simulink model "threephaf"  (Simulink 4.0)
settings: Solver=ode23  StartTime=-eps  StopTime=0.1  FixedStep=0.000001  MaxStep=2e-5  RelTol=1e-3
undefined symbols (not defined in the file or in its folder): Cdc, di, Element, L, R, sfunxy, Symmetrized, Tf, Ts, Udc, Upp, Warning, Yes
libraries: simulink3 x7
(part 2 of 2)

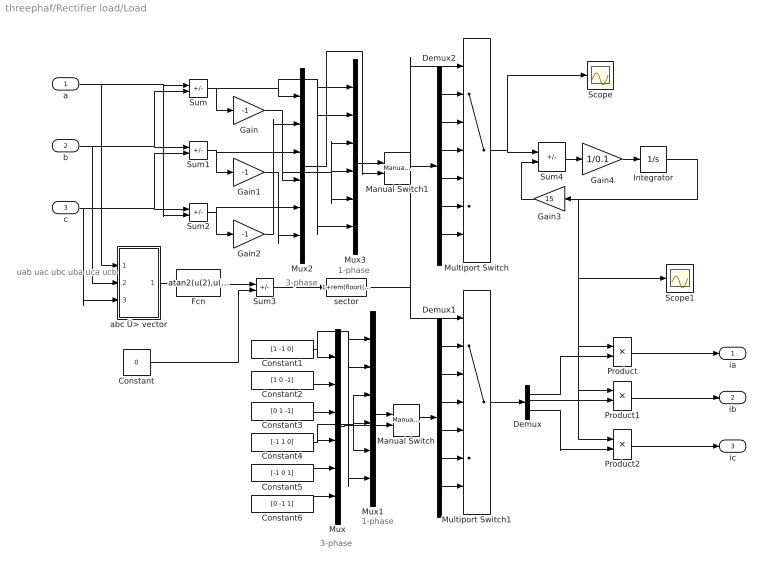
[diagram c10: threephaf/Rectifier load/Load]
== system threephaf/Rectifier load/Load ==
  note: uab uac ubc uba uca ucb
  note: 1-phase
  note: 3-phase
  note: 3-phase
  note: 1-phase
  a : Inport  Port=1  PortDimensions=-1  SampleTime=-1  DataType=auto
  b : Inport  Port=2  PortDimensions=-1  SampleTime=-1  DataType=auto
  c : Inport  Port=3  PortDimensions=-1  SampleTime=-1  DataType=auto
  Constant : Constant  Value=0
  Constant1 : Constant  Value=[1 -1 0]
  Constant2 : Constant  Value=[1 0 -1]
  Constant3 : Constant  Value=[0 1 -1]
  Constant4 : Constant  Value=[-1 1 0]
  Constant5 : Constant  Value=[-1 0 1]
  Constant6 : Constant  Value=[0 -1 1]
  Demux : Demux  Outputs=3  BusSelectionMode=off
  Demux1 : Demux  Outputs=6  BusSelectionMode=off
  Demux2 : Demux  Outputs=6  BusSelectionMode=off
  Fcn : Fcn  Expr=atan2(u(2),u(1))
  Gain : Gain  Gain=-1  Multiplication=Element-wise(K.*u)  SaturateOnIntegerOverflow=on
  Gain1 : Gain  Gain=-1  Multiplication=Element-wise(K.*u)  SaturateOnIntegerOverflow=on
  Gain2 : Gain  Gain=-1  Multiplication=Element-wise(K.*u)  SaturateOnIntegerOverflow=on
  Gain3 : Gain  Orientation=left  Gain=15  Multiplication=Element-wise(K.*u)  SaturateOnIntegerOverflow=on
  Gain4 : Gain  Gain=1/0.1  Multiplication=Element-wise(K.*u)  SaturateOnIntegerOverflow=on
  Integrator : Integrator  ExternalReset=none  InitialConditionSource=internal  InitialCondition=400*sqrt(2)*3/pi/50  LimitOutput=off  UpperSaturationLimit=inf  LowerSaturationLimit=-inf  ShowSaturationPort=off  ShowStatePort=off  AbsoluteTolerance=auto
  Manual Switch : simulink3/Nonlinear/Manual Switch  sw=0  action=0
  Manual Switch1 : simulink3/Nonlinear/Manual Switch  sw=0  action=0
  Multiport Switch : MultiPortSwitch  Inputs=6
  Multiport Switch1 : MultiPortSwitch  Inputs=6
  Mux{,1..3} (4 alike) : Mux  Inputs=6
  Product : Product  Inputs=2  Multiplication=Element-wise(.*)  SaturateOnIntegerOverflow=on
  Product1 : Product  Inputs=2  Multiplication=Element-wise(.*)  SaturateOnIntegerOverflow=on
  Product2 : Product  Inputs=2  Multiplication=Element-wise(.*)  SaturateOnIntegerOverflow=on
  Scope : Scope
  Scope1 : Scope
  Sum{,1..4} (5 alike) : Sum  Inputs=+-  SaturateOnIntegerOverflow=on
  abc Ü> vector : Subsystem  SimViewingDevice=off
  sector : Fcn  Expr=1+rem(floor((2*pi+u(1)+pi/3)/(pi/3+eps)),6)
  ia : Outport  Port=1  InitialOutput=0
  ib : Outport  Port=2  InitialOutput=0
  ic : Outport  Port=3  InitialOutput=0
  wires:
  Demux/3 -> Product2/2
  Demux/1 -> Product/2
  a/1 -> Sum/1, Sum2/2, abc Ü> vector/1(a)
  b/1 -> Sum1/1, Sum/2, abc Ü> vector/2(b)
  c/1 -> Sum2/1, Sum1/2, abc Ü> vector/3(c)
  Sum/1 -> Mux2/1, Mux3/2, Mux3/6, Mux3/1, Gain/1
  Sum1/1 -> Gain1/1, Mux2/3
  Sum2/1 -> Gain2/1, Mux2/5
  abc Ü> vector/1(vect) -> Fcn/1
  sector/1 -> Multiport Switch/1, Multiport Switch1/1
  Fcn/1 -> Sum3/1
  Sum3/1 -> sector/1
  Constant/1 -> Sum3/2
  Multiport Switch/1 -> Sum4/1, Scope/1
  Gain4/1 -> Integrator/1
  Gain3/1 -> Sum4/2
  Multiport Switch1/1 -> Demux/1
  Demux/2 -> Product1/2
  Product/1 -> ia/1
  Product1/1 -> ib/1
  Product2/1 -> ic/1
  Sum4/1 -> Gain4/1
  Integrator/1 -> Gain3/1, Product/1, Product1/1, Product2/1, Scope1/1
  Demux1/1 -> Multiport Switch1/2
  Demux1/2 -> Multiport Switch1/3
  Demux1/3 -> Multiport Switch1/4
  Demux1/4 -> Multiport Switch1/5
  Demux1/5 -> Multiport Switch1/6
  Demux1/6 -> Multiport Switch1/7
  Constant1/1 -> Mux/1, Mux1/2, Mux1/6, Mux1/1
  Constant2/1 -> Mux/2
  Constant3/1 -> Mux/3
  Constant4/1 -> Mux1/3, Mux1/4, Mux1/5, Mux/4
  Constant5/1 -> Mux/5
  Constant6/1 -> Mux/6
  Mux/1 -> Manual Switch/2
  Manual Switch/1 -> Demux1/1
  Mux1/1 -> Manual Switch/1
  Gain/1 -> Mux2/4, Mux3/3, Mux3/5, Mux3/4
  Gain1/1 -> Mux2/6
  Gain2/1 -> Mux2/2
  Demux2/1 -> Multiport Switch/2
  Demux2/2 -> Multiport Switch/3
  Demux2/3 -> Multiport Switch/4
  Demux2/4 -> Multiport Switch/5
  Demux2/5 -> Multiport Switch/6
  Demux2/6 -> Multiport Switch/7
  Mux3/1 -> Manual Switch1/1
  Manual Switch1/1 -> Demux2/1
  Mux2/1 -> Manual Switch1/2

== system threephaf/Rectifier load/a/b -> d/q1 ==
  vect : Inport  Port=1  PortDimensions=-1  SampleTime=-1  DataType=auto
  angle : Inport  Port=2  PortDimensions=-1  SampleTime=-1  DataType=auto
  Fcn_x : Fcn  Expr=u[1]*cos(u[3])-u[2]*sin(u[3])
  Fcn_y : Fcn  Expr=u[1]*sin(u[3])+u[2]*cos(u[3])
  Mux : Mux  Inputs=2
  Mux1 : Mux  Inputs=2
  Out : Outport  Port=1  InitialOutput=0
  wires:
  Mux1/1 -> Out/1
  Fcn_y/1 -> Mux1/2
  Fcn_x/1 -> Mux1/1
  Mux/1 -> Fcn_y/1, Fcn_x/1
  angle/1 -> Mux/2
  vect/1 -> Mux/1

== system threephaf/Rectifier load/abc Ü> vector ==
  a : Inport  Port=1  PortDimensions=-1  SampleTime=-1  DataType=auto
  b : Inport  Port=2  PortDimensions=-1  SampleTime=-1  DataType=auto
  c : Inport  Port=3  PortDimensions=-1  SampleTime=-1  DataType=auto
  Fcn : Fcn  Expr=sqrt(3/2)*u[1]
  Fcn1 : Fcn  Expr=sqrt(1/2)*(u[1]-u[2])
  Gain : Gain  Gain=1/3  Multiplication=Element-wise(K.*u)  SaturateOnIntegerOverflow=on
  Mux5 : Mux  Inputs=2
  Mux7 : Mux  Inputs=2
  Sum2 : Sum  Inputs=+++  SaturateOnIntegerOverflow=on
  Ü> ua : Sum  Inputs=+-  SaturateOnIntegerOverflow=on
  Ü> ub : Sum  Inputs=+-  SaturateOnIntegerOverflow=on
  Ü> uc : Sum  Inputs=+-  SaturateOnIntegerOverflow=on
  vect : Outport  Port=1  InitialOutput=0
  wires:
  Fcn1/1 -> Mux5/2
  Fcn/1 -> Mux5/1
  Mux5/1 -> vect/1
  Mux7/1 -> Fcn1/1
  Ü> uc/1 -> Mux7/2
  Ü> ub/1 -> Mux7/1
  Ü> ua/1 -> Fcn/1
  Gain/1 -> Ü> uc/2, Ü> ub/2, Ü> ua/2
  a/1 -> Ü> ua/1, Sum2/1
  b/1 -> Ü> ub/1, Sum2/2
  Sum2/1 -> Gain/1
  c/1 -> Ü> uc/1, Sum2/3

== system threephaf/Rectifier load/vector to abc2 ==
  vect : Inport  Port=1  PortDimensions=-1  SampleTime=-1  DataType=auto
  Ü> a : Fcn  Expr=sqrt(2/3)*u[1]
  Ü> b : Fcn  Expr=-sqrt(1/6)*u[1]+sqrt(1/2)*u[2]
  Ü> c : Fcn  Expr=-sqrt(1/6)*u[1]-sqrt(1/2)*u[2]
  a : Outport  Port=1  InitialOutput=0
  b : Outport  Port=2  InitialOutput=0
  c : Outport  Port=3  InitialOutput=0
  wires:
  vect/1 -> Ü> b/1, Ü> a/1, Ü> c/1
  Ü> b/1 -> b/1
  Ü> c/1 -> c/1
  Ü> a/1 -> a/1

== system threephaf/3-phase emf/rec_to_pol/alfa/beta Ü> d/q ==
  vect : Inport  Port=1  PortDimensions=-1  SampleTime=-1  DataType=auto
  angle : Inport  Port=2  PortDimensions=-1  SampleTime=-1  DataType=auto
  Fcn : Fcn  Expr=u[1]*cos(u[3])-u[2]*sin(u[3])
  Fcn1 : Fcn  Expr=u[1]*sin(u[3])+u[2]*cos(u[3])
  Mux : Mux  Inputs=2
  Mux1 : Mux  Inputs=2
  Out : Outport  Port=1  InitialOutput=0
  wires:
  vect/1 -> Mux/1
  angle/1 -> Mux/2
  Mux/1 -> Fcn/1, Fcn1/1
  Fcn/1 -> Mux1/1
  Fcn1/1 -> Mux1/2
  Mux1/1 -> Out/1

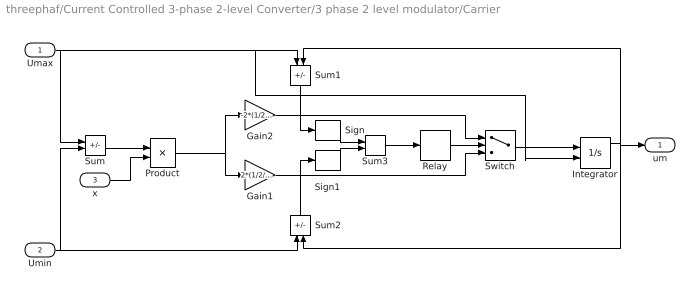
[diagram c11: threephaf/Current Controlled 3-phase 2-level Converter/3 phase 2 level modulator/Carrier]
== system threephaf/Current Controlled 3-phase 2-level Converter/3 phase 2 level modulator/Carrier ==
  Umax : Inport  Port=1  PortDimensions=-1  SampleTime=-1  DataType=auto
  Umin : Inport  Port=2  PortDimensions=-1  SampleTime=-1  DataType=auto
  x : Inport  Port=3  PortDimensions=-1  SampleTime=-1  DataType=auto
  Gain1 : Gain  Gain=2*(1/2/Ts)  Multiplication=Element-wise(K.*u)  SaturateOnIntegerOverflow=on
  Gain2 : Gain  Gain=-2*(1/2/Ts)  Multiplication=Element-wise(K.*u)  SaturateOnIntegerOverflow=on
  Integrator : Integrator  ExternalReset=none  InitialConditionSource=external  InitialCondition=0  LimitOutput=off  UpperSaturationLimit=inf  LowerSaturationLimit=-inf  ShowSaturationPort=off  ShowStatePort=off  AbsoluteTolerance=auto
  Product : Product  Inputs=2  Multiplication=Element-wise(.*)  SaturateOnIntegerOverflow=on
  Relay : Relay  OnSwitchValue=1  OffSwitchValue=-1  OnOutputValue=1  OffOutputValue=-1
  Sign : Signum
  Sign1 : Signum
  Sum : Sum  Inputs=+-  SaturateOnIntegerOverflow=on
  Sum1 : Sum  Orientation=down  Inputs=-+  SaturateOnIntegerOverflow=on
  Sum2 : Sum  Orientation=up  Inputs=-+  SaturateOnIntegerOverflow=on
  Sum3 : Sum  Inputs=++  SaturateOnIntegerOverflow=on
  Switch : Switch  Threshold=0
  um : Outport  Port=1
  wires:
  Switch/1 -> Integrator/1
  Umax/1 -> Sum/1, Sum1/1, Integrator/2
  Umin/1 -> Sum/2, Sum2/1
  Gain2/1 -> Switch/1
  Gain1/1 -> Switch/3
  Integrator/1 -> Sum1/2, um/1, Sum2/2
  Sum1/1 -> Sign/1
  Sum2/1 -> Sign1/1
  Sign/1 -> Sum3/1
  Sign1/1 -> Sum3/2
  Sum3/1 -> Relay/1
  Relay/1 -> Switch/2
  Sum/1 -> Product/1
  Product/1 -> Gain2/1, Gain1/1
  x/1 -> Product/2

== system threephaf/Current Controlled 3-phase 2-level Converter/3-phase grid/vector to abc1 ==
  vect : Inport  Port=1  PortDimensions=-1  SampleTime=-1  DataType=auto
  Ü> a : Fcn  Expr=sqrt(2/3)*u[1]
  Ü> b : Fcn  Expr=-sqrt(1/6)*u[1]+sqrt(1/2)*u[2]
  Ü> c : Fcn  Expr=-sqrt(1/6)*u[1]-sqrt(1/2)*u[2]
  a : Outport  Port=1  InitialOutput=0
  b : Outport  Port=2  InitialOutput=0
  c : Outport  Port=3  InitialOutput=0
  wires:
  vect/1 -> Ü> b/1, Ü> a/1, Ü> c/1
  Ü> b/1 -> b/1
  Ü> c/1 -> c/1
  Ü> a/1 -> a/1

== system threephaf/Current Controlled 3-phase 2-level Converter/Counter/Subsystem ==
  Trigger : TriggerPort  TriggerType=either  OutputDataType=auto
  Constant : Constant  Value=1
  Memory : Memory  Orientation=left  X0=0  InheritSampleTime=on
  Sum : Sum  Inputs=++  SaturateOnIntegerOverflow=on
  Out1 : Outport  Port=1
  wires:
  Sum/1 -> Memory/1, Out1/1
  Memory/1 -> Sum/2
  Constant/1 -> Sum/1

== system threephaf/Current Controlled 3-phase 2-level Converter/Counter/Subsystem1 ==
  Trigger : TriggerPort  TriggerType=either  OutputDataType=auto
  Constant : Constant  Value=1
  Memory : Memory  Orientation=left  X0=0  InheritSampleTime=on
  Sum : Sum  Inputs=++  SaturateOnIntegerOverflow=on
  Out1 : Outport  Port=1
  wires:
  Constant/1 -> Sum/1
  Memory/1 -> Sum/2
  Sum/1 -> Memory/1, Out1/1

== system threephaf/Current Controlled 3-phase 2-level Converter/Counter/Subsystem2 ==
  Trigger : TriggerPort  TriggerType=either  OutputDataType=auto
  Constant : Constant  Value=1
  Memory : Memory  Orientation=left  X0=0  InheritSampleTime=on
  Sum : Sum  Inputs=++  SaturateOnIntegerOverflow=on
  Out1 : Outport  Port=1
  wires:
  Sum/1 -> Memory/1, Out1/1
  Memory/1 -> Sum/2
  Constant/1 -> Sum/1

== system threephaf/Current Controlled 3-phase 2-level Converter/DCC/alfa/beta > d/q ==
  vect : Inport  Port=1  PortDimensions=-1  SampleTime=-1  DataType=auto
  angle : Inport  Port=2  PortDimensions=-1  SampleTime=-1  DataType=auto
  Fcn : Fcn  Expr=u[1]*cos(u[3])-u[2]*sin(u[3])
  Fcn1 : Fcn  Expr=u[1]*sin(u[3])+u[2]*cos(u[3])
  Mux : Mux  Inputs=2
  Mux1 : Mux  Inputs=2
  Out : Outport  Port=1  InitialOutput=0
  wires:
  vect/1 -> Mux/1
  angle/1 -> Mux/2
  Mux/1 -> Fcn/1, Fcn1/1
  Fcn/1 -> Mux1/1
  Fcn1/1 -> Mux1/2
  Mux1/1 -> Out/1

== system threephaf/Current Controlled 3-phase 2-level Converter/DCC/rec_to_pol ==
  rect : Inport  Port=1  PortDimensions=-1  SampleTime=-1  DataType=auto
  Derivative : Derivative
  Gain : Gain  Gain=-1  Multiplication=Element-wise(K.*u)  SaturateOnIntegerOverflow=on
  alfa/beta Ü> d/q : Subsystem  SimViewingDevice=off
  "angle " : Fcn  Expr=atan2(u[2],u[1])
  "mod " : Fcn  Expr=sqrt(u[1]^2+u[2]^2)
  mod : Outport  Port=1  InitialOutput=0
  angle : Outport  Port=2  InitialOutput=0
  emf : Outport  Port=3  InitialOutput=0
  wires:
  "angle "/1 -> angle/1, Gain/1
  rect/1 -> "angle "/1, "mod "/1, Derivative/1
  "mod "/1 -> mod/1
  Gain/1 -> alfa/beta Ü> d/q/2(angle)
  Derivative/1 -> alfa/beta Ü> d/q/1(vect)
  alfa/beta Ü> d/q/1(Out) -> emf/1

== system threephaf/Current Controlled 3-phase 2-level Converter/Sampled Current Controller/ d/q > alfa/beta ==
  vect : Inport  Port=1  PortDimensions=-1  SampleTime=-1  DataType=auto
  angle : Inport  Port=2  PortDimensions=-1  SampleTime=-1  DataType=auto
  Fcn : Fcn  Expr=u[1]*cos(u[3])-u[2]*sin(u[3])
  Fcn1 : Fcn  Expr=u[1]*sin(u[3])+u[2]*cos(u[3])
  Mux : Mux  Inputs=2
  Mux1 : Mux  Inputs=2
  Out : Outport  Port=1  InitialOutput=0
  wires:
  Mux1/1 -> Out/1
  Fcn1/1 -> Mux1/2
  Fcn/1 -> Mux1/1
  Mux/1 -> Fcn1/1, Fcn/1
  angle/1 -> Mux/2
  vect/1 -> Mux/1

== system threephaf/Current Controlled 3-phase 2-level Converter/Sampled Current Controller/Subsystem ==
  u : Inport  Orientation=left  Port=1  PortDimensions=-1  SampleTime=-1  DataType=auto
  Gammalt mätvärde2 : UnitDelay  Orientation=down  X0=0  SampleTime=Ts
  Gammalt mätvärde3 : UnitDelay  Orientation=left  X0=0  SampleTime=Ts
  Matsprediktor1 : Sum  Orientation=left  Inputs=+-  SaturateOnIntegerOverflow=on
  Proportional3 : Gain  Orientation=left  Gain=Ts/L  Multiplication=Element-wise(K.*u)  SaturateOnIntegerOverflow=on
  Proportional4 : Gain  Orientation=left  Gain=(1-Ts/(L/R))  Multiplication=Element-wise(K.*u)  SaturateOnIntegerOverflow=on
  Sum1 : Sum  Orientation=left  Inputs=++  SaturateOnIntegerOverflow=on
  di_smith : Outport  Orientation=left  Port=1
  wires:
  Proportional3/1 -> Sum1/1
  Proportional4/1 -> Sum1/2
  Sum1/1 -> Gammalt mätvärde2/1, Matsprediktor1/1
  u/1 -> Proportional3/1
  Matsprediktor1/1 -> Gammalt mätvärde3/1
  Gammalt mätvärde3/1 -> di_smith/1
  Gammalt mätvärde2/1 -> Proportional4/1, Matsprediktor1/2

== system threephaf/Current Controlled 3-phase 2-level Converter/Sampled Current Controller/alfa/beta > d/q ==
  vect : Inport  Port=1  PortDimensions=-1  SampleTime=-1  DataType=auto
  angle : Inport  Port=2  PortDimensions=-1  SampleTime=-1  DataType=auto
  Fcn : Fcn  Expr=u[1]*cos(u[3])-u[2]*sin(u[3])
  Fcn1 : Fcn  Expr=u[1]*sin(u[3])+u[2]*cos(u[3])
  Mux : Mux  Inputs=2
  Mux1 : Mux  Inputs=2
  Out : Outport  Port=1  InitialOutput=0
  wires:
  vect/1 -> Mux/1
  angle/1 -> Mux/2
  Mux/1 -> Fcn/1, Fcn1/1
  Fcn/1 -> Mux1/1
  Fcn1/1 -> Mux1/2
  Mux1/1 -> Out/1

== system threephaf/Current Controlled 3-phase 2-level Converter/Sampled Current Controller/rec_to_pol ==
  rect : Inport  Port=1  PortDimensions=-1  SampleTime=-1  DataType=auto
  Derivative : Derivative
  Gain : Gain  Gain=-1  Multiplication=Element-wise(K.*u)  SaturateOnIntegerOverflow=on
  alfa/beta Ü> d/q : Subsystem  SimViewingDevice=off
  "angle " : Fcn  Expr=atan2(u[2],u[1])
  "mod " : Fcn  Expr=sqrt(u[1]^2+u[2]^2)
  e : Outport  Port=1  InitialOutput=0
  angle : Outport  Port=2  InitialOutput=0
  mod : Outport  Port=3  InitialOutput=0
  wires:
  "angle "/1 -> angle/1, Gain/1
  rect/1 -> "angle "/1, "mod "/1, Derivative/1
  "mod "/1 -> mod/1
  Gain/1 -> alfa/beta Ü> d/q/2(angle)
  Derivative/1 -> alfa/beta Ü> d/q/1(vect)
  alfa/beta Ü> d/q/1(Out) -> e/1

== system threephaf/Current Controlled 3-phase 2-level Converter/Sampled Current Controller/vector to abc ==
  vect : Inport  Port=1  PortDimensions=-1  SampleTime=-1  DataType=auto
  Ü> a : Fcn  Expr=sqrt(2/3)*u[1]
  Ü> b : Fcn  Expr=-sqrt(1/6)*u[1]+sqrt(1/2)*u[2]
  Ü> c : Fcn  Expr=-sqrt(1/6)*u[1]-sqrt(1/2)*u[2]
  a : Outport  Port=1  InitialOutput=0
  b : Outport  Port=2  InitialOutput=0
  c : Outport  Port=3  InitialOutput=0
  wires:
  vect/1 -> Ü> b/1, Ü> a/1, Ü> c/1
  Ü> b/1 -> b/1
  Ü> c/1 -> c/1
  Ü> a/1 -> a/1

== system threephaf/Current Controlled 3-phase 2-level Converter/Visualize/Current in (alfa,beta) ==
  xy : Inport  Port=1  PortDimensions=-1  SampleTime=-1  DataType=auto
  sfunxy : S-Function  FunctionName=sfunxy  Parameters=[xmin xmax ymin ymax], st  PortCounts=[]  SFunctionModules=''
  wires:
  xy/1 -> sfunxy/1

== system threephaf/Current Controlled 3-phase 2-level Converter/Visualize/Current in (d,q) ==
  xy : Inport  Port=1  PortDimensions=-1  SampleTime=-1  DataType=auto
  sfunxy : S-Function  FunctionName=sfunxy  Parameters=[xmin xmax ymin ymax], st  PortCounts=[]  SFunctionModules=''
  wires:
  xy/1 -> sfunxy/1

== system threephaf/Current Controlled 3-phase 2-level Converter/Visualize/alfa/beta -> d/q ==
  vect : Inport  Port=1  PortDimensions=-1  SampleTime=-1  DataType=auto
  angle : Inport  Port=2  PortDimensions=-1  SampleTime=-1  DataType=auto
  Fcn : Fcn  Expr=u[1]*cos(u[3])-u[2]*sin(u[3])
  Fcn1 : Fcn  Expr=u[1]*sin(u[3])+u[2]*cos(u[3])
  Mux : Mux  Inputs=2
  Mux1 : Mux  Inputs=2
  Out : Outport  Port=1  InitialOutput=0
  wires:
  vect/1 -> Mux/1
  angle/1 -> Mux/2
  Mux/1 -> Fcn/1, Fcn1/1
  Fcn/1 -> Mux1/1
  Fcn1/1 -> Mux1/2
  Mux1/1 -> Out/1

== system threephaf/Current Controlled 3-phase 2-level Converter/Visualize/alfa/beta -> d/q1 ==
  vect : Inport  Port=1  PortDimensions=-1  SampleTime=-1  DataType=auto
  angle : Inport  Port=2  PortDimensions=-1  SampleTime=-1  DataType=auto
  Fcn : Fcn  Expr=u[1]*cos(u[3])-u[2]*sin(u[3])
  Fcn1 : Fcn  Expr=u[1]*sin(u[3])+u[2]*cos(u[3])
  Mux : Mux  Inputs=2
  Mux1 : Mux  Inputs=2
  Out : Outport  Port=1  InitialOutput=0
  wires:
  Mux1/1 -> Out/1
  Fcn1/1 -> Mux1/2
  Fcn/1 -> Mux1/1
  Mux/1 -> Fcn1/1, Fcn/1
  angle/1 -> Mux/2
  vect/1 -> Mux/1

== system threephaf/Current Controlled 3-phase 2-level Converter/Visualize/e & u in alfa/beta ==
  xy : Inport  Port=1  PortDimensions=-1  SampleTime=-1  DataType=auto
  sfunxy : S-Function  FunctionName=sfunxy4  Parameters=[xmin xmax ymin ymax], st  PortCounts=[]  SFunctionModules=''
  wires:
  xy/1 -> sfunxy/1

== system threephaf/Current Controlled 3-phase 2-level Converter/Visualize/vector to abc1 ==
  vect : Inport  Port=1  PortDimensions=-1  SampleTime=-1  DataType=auto
  Ü> a : Fcn  Expr=sqrt(2/3)*u[1]
  Ü> b : Fcn  Expr=-sqrt(1/6)*u[1]+sqrt(1/2)*u[2]
  Ü> c : Fcn  Expr=-sqrt(1/6)*u[1]-sqrt(1/2)*u[2]
  a : Outport  Port=1  InitialOutput=0
  b : Outport  Port=2  InitialOutput=0
  c : Outport  Port=3  InitialOutput=0
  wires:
  Ü> a/1 -> a/1
  Ü> c/1 -> c/1
  Ü> b/1 -> b/1
  vect/1 -> Ü> c/1, Ü> a/1, Ü> b/1

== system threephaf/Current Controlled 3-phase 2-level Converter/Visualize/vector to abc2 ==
  vect : Inport  Port=1  PortDimensions=-1  SampleTime=-1  DataType=auto
  Ü> a : Fcn  Expr=sqrt(2/3)*u[1]
  Ü> b : Fcn  Expr=-sqrt(1/6)*u[1]+sqrt(1/2)*u[2]
  Ü> c : Fcn  Expr=-sqrt(1/6)*u[1]-sqrt(1/2)*u[2]
  a : Outport  Port=1  InitialOutput=0
  b : Outport  Port=2  InitialOutput=0
  c : Outport  Port=3  InitialOutput=0
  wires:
  vect/1 -> Ü> b/1, Ü> a/1, Ü> c/1
  Ü> b/1 -> b/1
  Ü> c/1 -> c/1
  Ü> a/1 -> a/1

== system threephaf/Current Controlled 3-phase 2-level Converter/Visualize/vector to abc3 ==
  vect : Inport  Port=1  PortDimensions=-1  SampleTime=-1  DataType=auto
  Ü> a : Fcn  Expr=sqrt(2/3)*u[1]
  Ü> b : Fcn  Expr=-sqrt(1/6)*u[1]+sqrt(1/2)*u[2]
  Ü> c : Fcn  Expr=-sqrt(1/6)*u[1]-sqrt(1/2)*u[2]
  a : Outport  Port=1  InitialOutput=0
  b : Outport  Port=2  InitialOutput=0
  c : Outport  Port=3  InitialOutput=0
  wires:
  Ü> a/1 -> a/1
  Ü> c/1 -> c/1
  Ü> b/1 -> b/1
  vect/1 -> Ü> c/1, Ü> a/1, Ü> b/1

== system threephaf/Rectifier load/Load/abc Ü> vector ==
  a : Inport  Port=1  PortDimensions=-1  SampleTime=-1  DataType=auto
  b : Inport  Port=2  PortDimensions=-1  SampleTime=-1  DataType=auto
  c : Inport  Port=3  PortDimensions=-1  SampleTime=-1  DataType=auto
  Fcn : Fcn  Expr=sqrt(3/2)*u[1]
  Fcn1 : Fcn  Expr=sqrt(1/2)*(u[1]-u[2])
  Gain : Gain  Gain=1/3  Multiplication=Element-wise(K.*u)  SaturateOnIntegerOverflow=on
  Mux5 : Mux  Inputs=2
  Mux7 : Mux  Inputs=2
  Sum2 : Sum  Inputs=+++  SaturateOnIntegerOverflow=on
  Ü> ua : Sum  Inputs=+-  SaturateOnIntegerOverflow=on
  Ü> ub : Sum  Inputs=+-  SaturateOnIntegerOverflow=on
  Ü> uc : Sum  Inputs=+-  SaturateOnIntegerOverflow=on
  vect : Outport  Port=1  InitialOutput=0
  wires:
  c/1 -> Sum2/3, Ü> uc/1
  Sum2/1 -> Gain/1
  b/1 -> Sum2/2, Ü> ub/1
  a/1 -> Sum2/1, Ü> ua/1
  Gain/1 -> Ü> ua/2, Ü> ub/2, Ü> uc/2
  Ü> ua/1 -> Fcn/1
  Ü> ub/1 -> Mux7/1
  Ü> uc/1 -> Mux7/2
  Mux7/1 -> Fcn1/1
  Mux5/1 -> vect/1
  Fcn/1 -> Mux5/1
  Fcn1/1 -> Mux5/2

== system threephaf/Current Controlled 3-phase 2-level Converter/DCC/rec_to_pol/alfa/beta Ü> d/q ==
  vect : Inport  Port=1  PortDimensions=-1  SampleTime=-1  DataType=auto
  angle : Inport  Port=2  PortDimensions=-1  SampleTime=-1  DataType=auto
  Fcn : Fcn  Expr=u[1]*cos(u[3])-u[2]*sin(u[3])
  Fcn1 : Fcn  Expr=u[1]*sin(u[3])+u[2]*cos(u[3])
  Mux : Mux  Inputs=2
  Mux1 : Mux  Inputs=2
  Out : Outport  Port=1  InitialOutput=0
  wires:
  vect/1 -> Mux/1
  angle/1 -> Mux/2
  Mux/1 -> Fcn/1, Fcn1/1
  Fcn/1 -> Mux1/1
  Fcn1/1 -> Mux1/2
  Mux1/1 -> Out/1

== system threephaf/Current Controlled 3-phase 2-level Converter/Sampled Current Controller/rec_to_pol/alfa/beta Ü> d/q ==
  vect : Inport  Port=1  PortDimensions=-1  SampleTime=-1  DataType=auto
  angle : Inport  Port=2  PortDimensions=-1  SampleTime=-1  DataType=auto
  Fcn : Fcn  Expr=u[1]*cos(u[3])-u[2]*sin(u[3])
  Fcn1 : Fcn  Expr=u[1]*sin(u[3])+u[2]*cos(u[3])
  Mux : Mux  Inputs=2
  Mux1 : Mux  Inputs=2
  Out : Outport  Port=1  InitialOutput=0
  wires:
  vect/1 -> Mux/1
  angle/1 -> Mux/2
  Mux/1 -> Fcn/1, Fcn1/1
  Fcn/1 -> Mux1/1
  Fcn1/1 -> Mux1/2
  Mux1/1 -> Out/1
